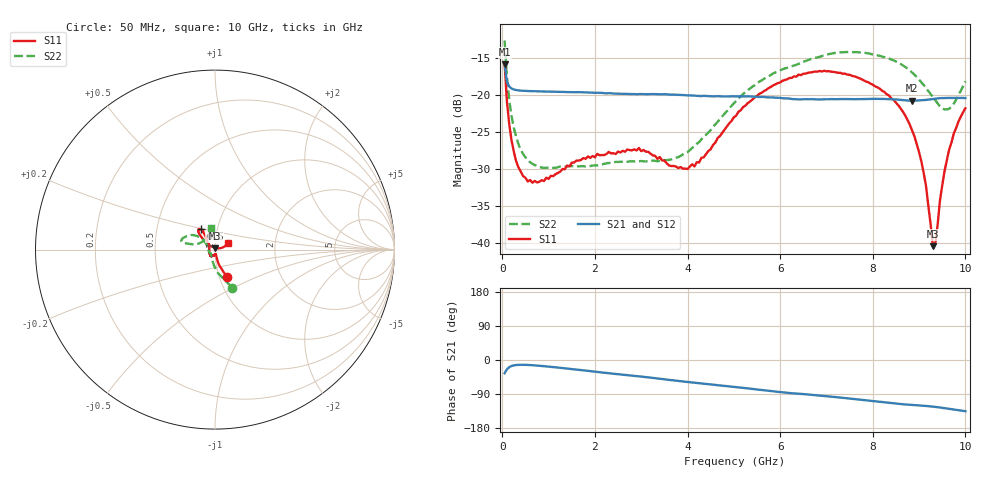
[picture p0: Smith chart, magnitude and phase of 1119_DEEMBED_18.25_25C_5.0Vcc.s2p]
!Hittite Microwave Corp.
!Digital Attenuator/PhaseShifter Rev 1.4.0
!Filename: C:\DATA\DATA\1119_DEEMBED_18.25_25C_5.0Vcc.s2p
!VNA ID: Agilent Technologies,N5224A,MY51441122,A.10.45.03
!Device type:
!2 Port Calibration.
!Temp(C): 25
!Lot Number:
!Serial Number:
!Operator:
!Misc:
!Attenuator:  18.250
# GHZ S DB R 50.0
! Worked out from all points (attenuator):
!   200 points, 50 MHz to 10 GHz, reference 50 ohm
!   highest |S21| = -15.87 dB at 50 MHz (marker M1); lowest = -20.8 dB at 8.85 GHz (marker M2)
!   lowest |S11| = -40.4 dB at 9.3 GHz (marker M3), VSWR 1.02, Z = 50 + j0.952 ohm
!   |S11| at or under -10 dB: start of sweep to end of sweep
!   |S22| runs from -29.9 to -12.7 dB; largest |S21 - S12| = 0.00034
!   S11 on the Smith chart (normalised r, x): 50 MHz: 1.08, -0.34; 6.5 GHz: 0.83, +0.19; 10 GHz: 1.15, +0.09
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0.05  -15.67 -66.8  -15.87 -34.9  -15.87 -35.0  -12.68 -65.7
0.1  -20.92 -74.9  -18.24 -24.6  -18.23 -24.6  -17.62 -82.9
0.2  -26.18 -78.1  -19.16 -15.8  -19.16 -15.8  -22.90 -99.7
0.45  -30.97 -78.4  -19.46 -12.6  -19.47 -12.6  -28.00 -120.1
0.9  -31.64 -88.6  -19.56 -16.3  -19.56 -16.3  -29.86 -134.2
1.75  -28.54 -110.4  -19.68 -27.2  -19.68 -27.2  -29.63 -138.6
2.95  -27.18 -125.8  -19.91 -43.1  -19.92 -43.1  -28.96 -157.6
3.4  -28.40 -143.6  -19.94 -49.4  -19.94 -49.5  -28.90 -170.9
4.15  -29.66 166.1  -20.11 -60.0  -20.13 -60.1  -26.93 158.5
5.05  -22.82 128.3  -20.22 -71.4  -20.24 -71.4  -20.84 140.2
5.75  -19.10 124.2  -20.35 -81.2  -20.37 -81.2  -17.50 144.4
6.5  -17.17 125.5  -20.62 -89.9  -20.63 -89.9  -15.56 152.5
6.7  -16.95 126.9  -20.60 -92.2  -20.61 -92.2  -15.11 154.9
7.5  -17.30 133.1  -20.59 -101.8  -20.60 -101.8  -14.24 164.0
8.35  -20.11 137.7  -20.60 -112.8  -20.60 -112.8  -15.12 167.8
8.85  -24.83 140.4  -20.80 -118.6  -20.80 -118.6  -17.01 167.3
9.15  -32.31 137.6  -20.70 -121.2  -20.71 -121.3  -19.09 164.6
9.3  -40.42 90.8  -20.58 -123.1  -20.60 -123.1  -20.32 159.3
9.35  -40.07 56.5  -20.54 -123.8  -20.56 -123.8  -20.75 156.4
9.45  -34.30 19.7  -20.46 -125.4  -20.48 -125.4  -21.54 148.9
9.65  -27.36 15.1  -20.43 -128.8  -20.44 -128.8  -21.88 127.0
10  -21.83 27.1  -20.45 -135.1  -20.45 -135.1  -18.19 99.7
